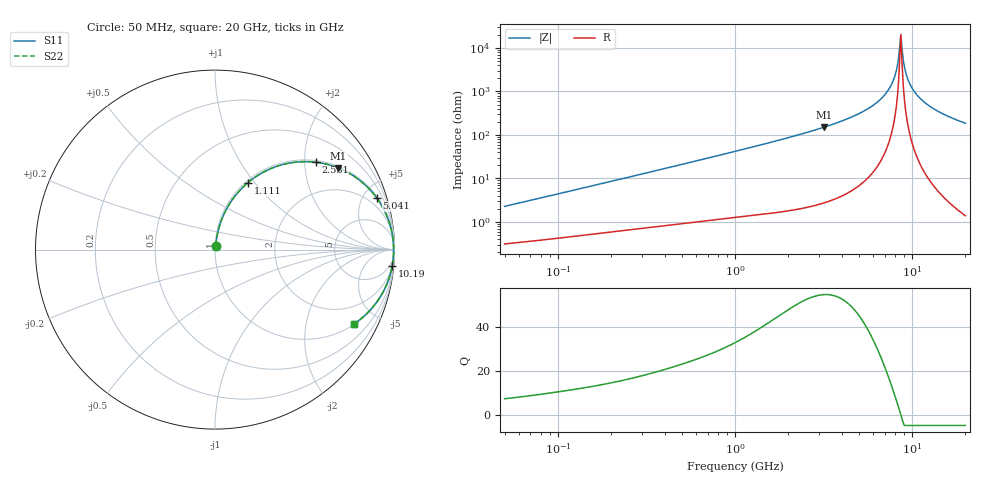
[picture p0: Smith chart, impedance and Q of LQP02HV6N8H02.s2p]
!Murata Part Number: LQP02HV6N8H02
!These Parameters are Measured in Series Mode Connection
!  o--[Z]--o
!Port1  Port2
!  o-------o
!Freq. Start=50[MHz] Stop=20[GHz], 401[Steps]
# Hz S RI R 50
!Freq.(Hz) S11(Real) S11(Imag) S21(Real) S21(Imag) S12(Real) S12(Imag) S22(Real) S22(Imag)
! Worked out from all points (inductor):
!   401 points, 50 MHz to 20 GHz, reference 50 ohm
!   read as one part in series: L = 7.09 nH near 51.52 MHz
!   highest Q = 55 at 3.169 GHz (marker M1), where L = 7.5 nH
!   self-resonance near 8.516 GHz
!   S11 on the Smith chart (normalised r, x): 50 MHz: 1.01, +0.05; 1.111 GHz: 1.03, +0.93; 2.531 GHz: 1.04, +2.26; 5.041 GHz: 1.14, +6.23; 10.19 GHz: 2, -21; 20 GHz: 1.03, -3.70
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5e7  0.00361 0.0224  0.9964 -0.0224  0.9964 -0.0224  0.00361 0.0224
1.364002e8  0.00828 0.0582  0.9917 -0.0582  0.9917 -0.0582  0.00828 0.0582
3.721004e8  0.0311 0.1504  0.9689 -0.1504  0.9689 -0.1504  0.0311 0.1504
1e9  0.1559 0.3479  0.8441 -0.3479  0.8441 -0.3479  0.1559 0.3479
1.110545e9  0.1843 0.3737  0.8157 -0.3737  0.8157 -0.3737  0.1843 0.3737
2.531158e9  0.56 0.487  0.44 -0.487  0.44 -0.487  0.56 0.487
2.728004e9  0.6029 0.4801  0.3971 -0.4801  0.3971 -0.4801  0.6029 0.4801
3.168813e9  0.6875 0.4545  0.3125 -0.4545  0.3125 -0.4545  0.6875 0.4545
5.041459e9  0.9015 0.2871  0.0985 -0.2871  0.0985 -0.2871  0.9015 0.2871
6.406762e9  0.9659 0.1654  0.0341 -0.1654  0.0341 -0.1654  0.9659 0.1654
7.442007e9  0.9877 0.0834  0.0123 -0.0834  0.0123 -0.0834  0.9877 0.0834
8.020766e9  0.9932 0.0415  0.00676 -0.0415  0.00676 -0.0415  0.9932 0.0415
8.141811e9  0.9939 0.0331  0.00609 -0.0331  0.00609 -0.0331  0.9939 0.0331
8.389408e9  0.9948 0.0163  0.00518 -0.0163  0.00518 -0.0163  0.9948 0.0163
8.644534e9  0.9952 -0.00061  0.00484 0.00061  0.00484 0.00061  0.9952 -0.00061
8.907419e9  0.9949 -0.0175  0.00508 0.0175  0.00508 0.0175  0.9949 -0.0175
9.041845e9  0.9946 -0.0259  0.00542 0.0259  0.00542 0.0259  0.9946 -0.0259
9.316812e9  0.9935 -0.0428  0.00653 0.0428  0.00653 0.0428  0.9935 -0.0428
1.019291e10  0.9867 -0.0931  0.0133 0.0931  0.0133 0.0931  0.9867 -0.0931
1.131968e10  0.9722 -0.151  0.0278 0.151  0.0278 0.151  0.9722 -0.151
1.314879e10  0.9391 -0.2307  0.0609 0.2307  0.0609 0.2307  0.9391 -0.2307
2e10  0.7727 -0.4154  0.2273 0.4154  0.2273 0.4154  0.7727 -0.4154
